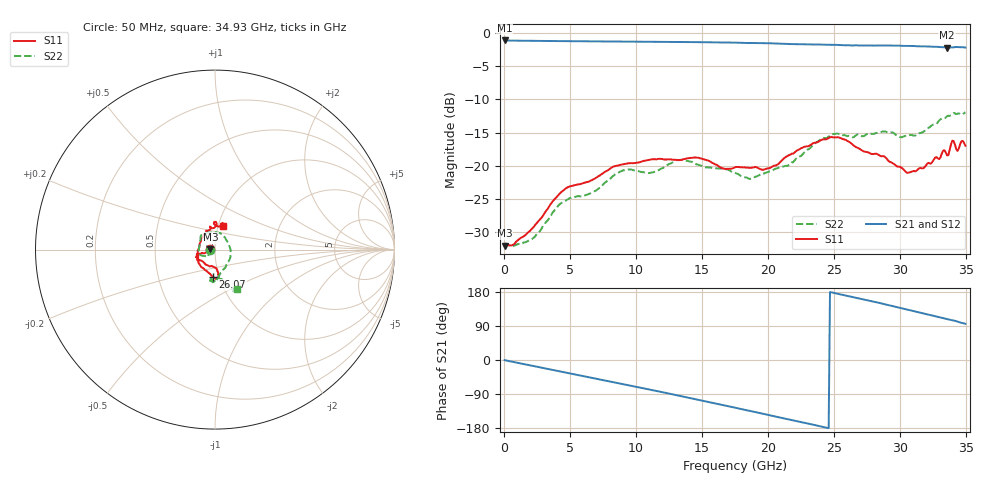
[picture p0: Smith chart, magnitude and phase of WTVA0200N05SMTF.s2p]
! 50 ohm 2-Port S-parameters measured by Modelithics Inc support@modelithics.com  Tampa, FL USA 813-866-6335 (February 2024)
! Smiths Interconnect,  2dB P/N: WTVA0200N05SMTF, Temperature: 125 C
! Board: 10 mil Rogers 4350B, Mounting Pad Dimensions: Length: 15 mils, Width: 25 mils, Gap: 40 mils.
# Hz S RI R 50
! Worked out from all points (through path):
!   352 points, 50 MHz to 34.93 GHz, reference 50 ohm
!   highest |S21| = -1.13 dB at 50 MHz (marker M1); lowest = -2.2 dB at 33.53 GHz (marker M2)
!   group delay of S21, straight-line fit = 20.9 ps
!   lowest |S11| = -32.0 dB at 50 MHz (marker M3), VSWR 1.05, Z = 47.5 + j0.111 ohm
!   |S11| at or under -10 dB: start of sweep to end of sweep
!   |S22| runs from -32.1 to -11.9 dB; largest |S21 - S12| = 0.0098
!   S11 on the Smith chart (normalised r, x): 50 MHz: 0.95, +0.00; 26.07 GHz: 0.93, -0.29; 34.93 GHz: 1.06, +0.29
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5e7  -0.0251 0.00117  0.8777 -0.00505  0.8765 -0.00501  -0.0251 0.000392
2.0905e9  -0.0332 -0.00466  0.8431 -0.2238  0.842 -0.224  -0.0269 -0.00811
4.18e9  -0.058 -0.02  0.7554 -0.4277  0.7539 -0.4273  -0.0381 -0.0342
5.8715e9  -0.0711 -0.0186  0.6492 -0.5724  0.6483 -0.5718  -0.0426 -0.0408
8.956e9  -0.0998 -0.024  0.3883 -0.7677  0.3869 -0.767  -0.0883 -0.0261
1.1742e10  -0.1053 -0.0416  0.1024 -0.85  0.1005 -0.8491  -0.0838 0.0418
1.3533e10  -0.0994 -0.0514  -0.0936 -0.8498  -0.0954 -0.8485  -0.0696 0.087
1.7513e10  -0.0555 -0.0807  -0.497 -0.6838  -0.4969 -0.6823  0.0515 0.072
1.86075e10  -0.036 -0.0897  -0.5858 -0.601  -0.5861 -0.5993  0.0731 0.0324
2.01e10  -0.00712 -0.096  -0.6905 -0.4713  -0.6897 -0.4702  0.0874 -0.025
2.33835e10  0.02 -0.1465  -0.8079 -0.1343  -0.8066 -0.1344  0.0245 -0.1412
2.47765e10  0.0159 -0.1642  -0.814 0.0199  -0.8127 0.0213  0.005 -0.1725
2.607e10  -0.0108 -0.1525  -0.7927 0.1588  -0.791 0.1595  -0.0195 -0.1673
2.91545e10  -0.0928 -0.055  -0.6541 0.4681  -0.6485 0.473  -0.000876 -0.1772
3.05475e10  -0.0879 0.0129  -0.543 0.5856  -0.5396 0.5871  0.0336 -0.166
3.29355e10  -0.0363 0.1066  -0.3037 0.7221  -0.2981 0.7229  0.0769 -0.2051
3.33335e10  -0.0285 0.1282  -0.2598 0.7358  -0.2554 0.7359  0.0824 -0.2128
3.35325e10  -0.0181 0.1188  -0.239 0.7363  -0.2331 0.7369  0.0892 -0.2187
3.39305e10  0.00442 0.1548  -0.1987 0.7521  -0.1929 0.7522  0.1048 -0.2217
3.43285e10  0.0182 0.1284  -0.1503 0.7683  -0.1458 0.7676  0.1079 -0.2221
3.4627e10  0.0428 0.1474  -0.1109 0.7738  -0.1107 0.7719  0.1074 -0.2181
3.49255e10  0.047 0.1338  -0.0745 0.7725  -0.0737 0.7707  0.1225 -0.2218
